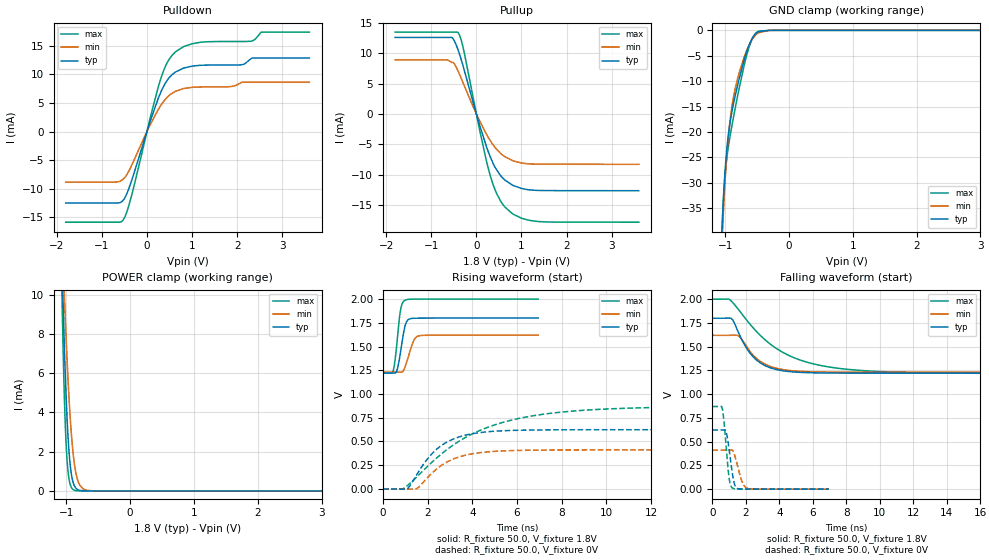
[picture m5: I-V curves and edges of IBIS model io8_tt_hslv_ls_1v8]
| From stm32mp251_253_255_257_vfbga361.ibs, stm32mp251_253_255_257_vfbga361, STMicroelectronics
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[Model]   io8_tt_hslv_ls_1v8
Model_type I/O
Polarity   Non-Inverting
Enable   Active-Low
| CAP_THRESHOLD on pad IOTT is "UDTCAPC" :
| Rising=30.0% of vddiov33m   Falling=70.0% of vddiov33m
| C_comp min and max val. don't necessarily correlate with the min and max pvt
| but are the smallest and greatest pad capacitance found.
| var   typ   min   max
C_comp   1.16083pF  1.09792pF  1.36396pF
|C_comp_pullup   764.88000fF  538.04000fF  521.01000fF
|C_comp_pulldown   395.95350fF  559.87540fF  842.95418fF
Vinl = 486.0mV
Vinh = 1.4V
Vmeas = 900.0mV   | Reference voltage for timing measurements
Cref  = 50.0pF   | Timing specification test load capacitance value
Rref  = 100.0MOhm   | Timing specification test load resistance value
Vref  = 900.0mV   | Timing specification test load voltage
[Model Spec]
| TIME_THRESHOLD on pin ZIV08M is "CMOS" :
| Rising=50.0% of vddv08m   Falling=50.0% of vddv08m
Vinl 675.70000mV 623.70000mV 735.70000mV
Vinh 1.12730V 1.01130V 1.24930V
| variable   typ   min   max
[Temperature Range] 25.0 125.0 -40.0
| variable   typ   min   max
[Voltage Range] 1.8V 1.62V 2.0V
| variable   typ   min   max
[POWER Clamp Reference] 1.8V 1.62V 2.0V
| variable   typ   min   max
[GND Clamp Reference] 0V 0V 0V
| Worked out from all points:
|   slope of the pulldown table from 0 to 0.27 V, typ, clamps not added: 43.9 ohm
|   slope of the pullup table from 0 to 0.27 V, typ, clamps not added: 42.7 ohm
|   GND clamp passes 1 mA (typ) near -0.55 V on its own axis
|   POWER clamp passes 1 mA (typ) near -0.93 V on its own axis
|   rising waveform, R_fixture 50.0, V_fixture 1.8V: 20-80 % time 245ps typ, 319ps min, 209ps max; typ from 1.22 V to 1.8 V
|   falling waveform, R_fixture 50.0, V_fixture 1.8V: 20-80 % time 1.33ns typ, 1.34ns min, 3.23ns max; typ from 1.8 V to 1.22 V
|   rising waveform, R_fixture 50.0, V_fixture 0V: 20-80 % time 1.46ns typ, 1.45ns min, 3.58ns max; typ from 0 V to 0.624 V
|   falling waveform, R_fixture 50.0, V_fixture 0V: 20-80 % time 299ps typ, 387ps min, 258ps max; typ from 0.624 V to 0 V
[POWER Clamp]
-1.8V     152.1mA    105.6mA    221.1mA
-1.07V    12.07mA    13.61mA    10.38mA
-1.05V    9.569mA    11.75mA    7.248mA
-1.03V    7.339mA    9.993mA    4.743mA
-1.01V    5.42mA     8.358mA    2.898mA
-990mV    3.841mA    6.859mA    1.662mA
-970mV    2.609mA    5.513mA    906.4uA
-940mV    1.358mA    3.806mA    344.1uA
-880mV    308.2uA    1.548mA    45.5uA
-790mV    28.46uA    298.9uA    2.106uA
-610mV    213nA      7.572uA    9.541nA
3.6V      0A         0A         0A
[GND Clamp]
-1.8V     -1.214A    -1.184A    -1.231A
-1.05V    -39.75mA   -42.57mA   -39.2mA
-1.04V    -36.64mA   -39.37mA   -36.3mA
-1.01V    -29.33mA   -31.48mA   -29.9mA
-970mV    -22.87mA   -23.87mA   -24.77mA
-920mV    -17.89mA   -17.43mA   -20.6mA
-870mV    -14.47mA   -13.19mA   -17.12mA
-780mV    -9.529mA   -8.318mA   -11.38mA
-650mV    -3.743mA   -3.579mA   -4.327mA
-570mV    -1.451mA   -1.665mA   -1.53mA
-490mV    -324.1uA   -556uA     -259.6uA
3.6V      61.92nA    2.591uA    17.99nA
| variable   typ   min   max
[Pullup Reference] 1.8V 1.62V 2.0V
| variable   typ   min   max
[Pulldown Reference] 0V 0V 0V
[Pullup]
-1.8V     12.57mA    8.892mA    13.45mA
-670mV    12.57mA    8.892mA    13.45mA
-540mV    12.57mA    8.457mA    13.45mA
-490mV    12.03mA    8.269mA    13.45mA
-390mV    10.19mA    6.794mA    13.18mA
-290mV    7.763mA    5.031mA    10.78mA
70mV      -1.782mA   -1.112mA   -2.559mA
320mV     -7.265mA   -4.527mA   -10.43mA
530mV     -10.07mA   -6.443mA   -14.24mA
810mV     -11.75mA   -7.702mA   -16.46mA
1.37V     -12.57mA   -8.252mA   -17.68mA
3.6V      -12.62mA   -8.28mA    -17.79mA
[Pulldown]
-1.8V     -12.46mA   -8.848mA   -15.82mA
-520mV    -11.93mA   -8.267mA   -15.35mA
-310mV    -7.858mA   -5.414mA   -10.27mA
70mV      1.735mA    1.162mA    2.316mA
290mV     6.538mA    4.344mA    8.798mA
450mV     8.944mA    5.975mA    12.02mA
630mV     10.37mA    7.006mA    13.9mA
1.18V     11.56mA    7.772mA    15.57mA
2.09V     11.64mA    8.541mA    15.71mA
2.32V     12.79mA    8.594mA    15.78mA
2.54V     12.82mA    8.594mA    17.35mA
3.6V      12.82mA    8.594mA    17.35mA
[Ramp]
dV/dt_r 374.37951mV/1.45582ns 246.68175mV/1.4499ns 522.26302mV/3.57881ns
dV/dt_f 347.16309mV/1.32919ns 233.37412mV/1.33676ns 468.15497mV/3.2246ns
R_load = 50.0
| Removed startup time: 0s 0s 0s  .
| Removed end time: 6.95ns.
[Rising Waveform]
R_fixture   = 50.0
V_fixture   = 1.8V
V_fixture_min = 1.62V
V_fixture_max = 2.0V
0s        1.222V     1.231V     1.22V
450ps     1.222V     1.231V     1.234V
600ps     1.23V      1.231V     1.476V
750ps     1.389V     1.231V     1.828V
800ps     1.462V     1.231V     1.904V
1ns       1.727V     1.293V     1.99V
1.1ns     1.776V     1.365V     1.996V
1.35ns    1.797V     1.547V     1.999V
1.6ns     1.799V     1.612V     1.999V
6.95ns    1.8V       1.62V      2V
| Removed startup time: 0s 0s 0s  .
| Removed end time: 34.9ns.
[Falling Waveform]
R_fixture   = 50.0
V_fixture   = 1.8V
V_fixture_min = 1.62V
V_fixture_max = 2.0V
0s        1.8V       1.62V      2V
1ns       1.801V     1.62V      2V
1.2ns     1.787V     1.621V     1.967V
1.6ns     1.631V     1.609V     1.881V
2.2ns     1.443V     1.46V      1.747V
3.2ns     1.296V     1.311V     1.564V
5ns       1.232V     1.244V     1.375V
7.5ns     1.222V     1.232V     1.273V
13.5ns    1.222V     1.231V     1.224V
34.9ns    1.222V     1.231V     1.22V
| Removed startup time: 0s 0s 0s  .
| Removed end time: 34.8ns.
[Rising Waveform]
R_fixture   = 50.0
V_fixture   = 0V
V_fixture_min = 0V
V_fixture_max = 0V
0s        0V         0V         0V
900ps     -1.691mV   -863.3uV   1.419mV
1.1ns     2.486mV    -1.111mV   36.83mV
1.5ns     144.8mV    1.783mV    123.4mV
2.2ns     372.4mV    168.3mV    283.1mV
3.4ns     547.6mV    336.7mV    501.6mV
5.4ns     613.1mV    401mV      703.3mV
7.9ns     622.9mV    410.2mV    807.2mV
13.9ns    623.8mV    411.1mV    863.9mV
34.8ns    623.8mV    411.1mV    870.3mV
| Removed startup time: 0s 0s 0s  .
| Removed end time: 6.95ns.
[Falling Waveform]
R_fixture   = 50.0
V_fixture   = 0V
V_fixture_min = 0V
V_fixture_max = 0V
0s        623.8mV    411.1mV    870.3mV
600ps     623.8mV    411.1mV    841.4mV
800ps     614.7mV    411.1mV    495mV
1ns       415.3mV    411mV      113.7mV
1.2ns     156.3mV    408.6mV    11.25mV
1.3ns     64.38mV    371.7mV    4.107mV
1.45ns    10.59mV    281.3mV    1.549mV
1.8ns     1.079mV    66.51mV    611.2uV
2.1ns     586.1uV    8.063mV    380.1uV
6.95ns    0V         0V         0V
